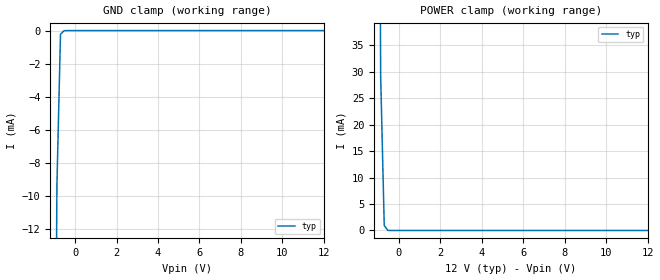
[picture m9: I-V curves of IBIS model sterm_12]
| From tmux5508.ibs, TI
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| sterm_12
[Model]   sterm_12
Model_type   Terminator
|   typ   min   max
C_comp   2.533030e-12   NA   NA
[Voltage Range]   12   NA   NA
[Temperature Range]   27   NA   NA
[Power Clamp Reference]   12   NA   NA
[GND Clamp Reference]   0   NA   NA
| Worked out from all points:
|   GND clamp passes 1 mA (typ) near -0.72 V on its own axis
|   POWER clamp passes 1 mA (typ) near -0.71 V on its own axis
[GND Clamp]
|   Voltage   I(typ)   I(min)   I(max)
-5V       -2.839A    NA         NA
-1.051V   -42.72mA   NA         NA
-878.8mV  -9.288mA   NA         NA
-707.1mV  -223.6uA   NA         NA
-535.4mV  -9.048uA   NA         NA
12V       1.089nA    NA         NA
[POWER Clamp]
|   Voltage   I(typ)   I(min)   I(max)
-5V       6.669A     NA         NA
-1.05V    166mA      NA         NA
-878.8mV  29.09mA    NA         NA
-707.1mV  960.6uA    NA         NA
-535.4mV  6.001uA    NA         NA
12V       -1.319nA   NA         NA
